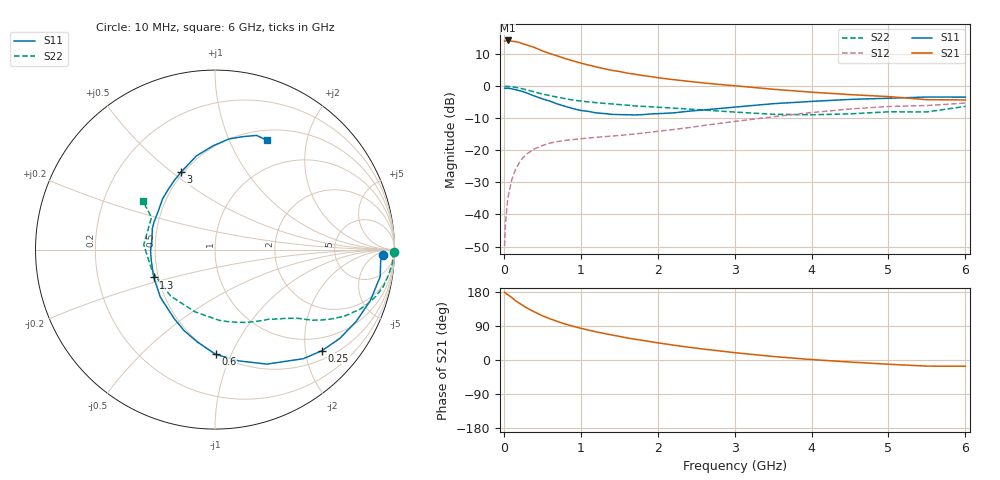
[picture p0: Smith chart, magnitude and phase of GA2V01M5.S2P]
! Infineon Technologies  Discrete & RF Semiconductors
! BF775
! Si NPN RF Bipolar Junction Transistor in SOT23
! VCE = 2 V  IC = 1.5 mA
! Common Emitter S-Parameters:  May  1996
# GHz  S  MA  R  50
!  f  S11  S21  S12  S22
! GHz  MAG  ANG  MAG  ANG  MAG  ANG  MAG  ANG
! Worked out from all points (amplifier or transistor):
!   36 points, 10 MHz to 6 GHz, reference 50 ohm
!   highest |S21| = 14.3 dB at 50 MHz (marker M1)
!   |S21| within 3 dB of that: start of sweep to 476 MHz
!   unconditionally stable (mu >= 1): 1.251 GHz to end of sweep
!   at 250 MHz: K = 0.25, MSG = 17.7 dB, |S12| = -22.3 dB
!   at 1.4 GHz: K = 1.08, MAG = 8.6 dB, |S12| = -15.6 dB
!   at 6 GHz: K = 1.03, MAG = -0.6 dB, |S12| = -5.3 dB
!   S11 on the Smith chart (normalised r, x): 10 MHz: 24, -11; 250 MHz: 0.68, -2.35; 600 MHz: 0.49, -0.87; 1.3 GHz: 0.47, -0.17; 3 GHz: 0.49, +0.54; 6 GHz: 0.62, +1.39
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0.01  0.9342 -1.8  5.048 178.9  0.0032 90.9  0.9993 -0.8
0.02  0.9252 -3.8  5.066 176.9  0.007 86.6  0.9911 -1.7
0.05  0.9325 -9.3  5.16 172.4  0.0172 84.7  0.9916 -4.3
0.1  0.9111 -18.1  5.034 165.2  0.0337 79.5  0.9763 -8.5
0.15  0.8825 -27.0  4.943 156.9  0.0499 73.6  0.9593 -12.5
0.2  0.8535 -35.4  4.806 150.1  0.0636 69.3  0.9334 -16.2
0.25  0.8204 -43.3  4.568 143.6  0.0768 64.5  0.9043 -19.4
0.3  0.7821 -51.0  4.383 137.2  0.088 60.9  0.875 -22.2
0.4  0.7006 -65.6  4.006 126.6  0.1055 54.2  0.8115 -27.2
0.5  0.6338 -78.0  3.548 116.8  0.1185 49.0  0.7533 -30.9
0.6  0.5834 -89.7  3.223 108.8  0.1296 45.1  0.7107 -33.5
0.8  0.4836 -110.8  2.69 94.8  0.143 40.0  0.6377 -37.6
0.9  0.4466 -120.6  2.478 88.9  0.1471 38.9  0.6069 -39.2
1.1  0.4037 -139.0  2.137 79.0  0.1556 37.2  0.5679 -42.4
1.3  0.3748 -155.6  1.875 70.3  0.1633 36.6  0.5396 -45.3
1.7  0.3557 173.0  1.538 55.0  0.1792 38.7  0.4921 -51.8
2.2  0.3825 145.4  1.265 39.4  0.2105 40.7  0.4549 -62.2
3  0.471 113.8  1.015 19.4  0.2815 39.9  0.395 -86.5
3.5  0.533 101.1  0.895 9.3  0.3336 36.2  0.3642 -107.7
4.5  0.6216 82.8  0.738 -5.4  0.4402 24.4  0.3697 -159.9
5.5  0.6772 70.0  0.615 -16.1  0.4987 8.7  0.3967 153.1
6  0.6743 64.5  0.61 -16.4  0.5448 4.3  0.4834 146.1
